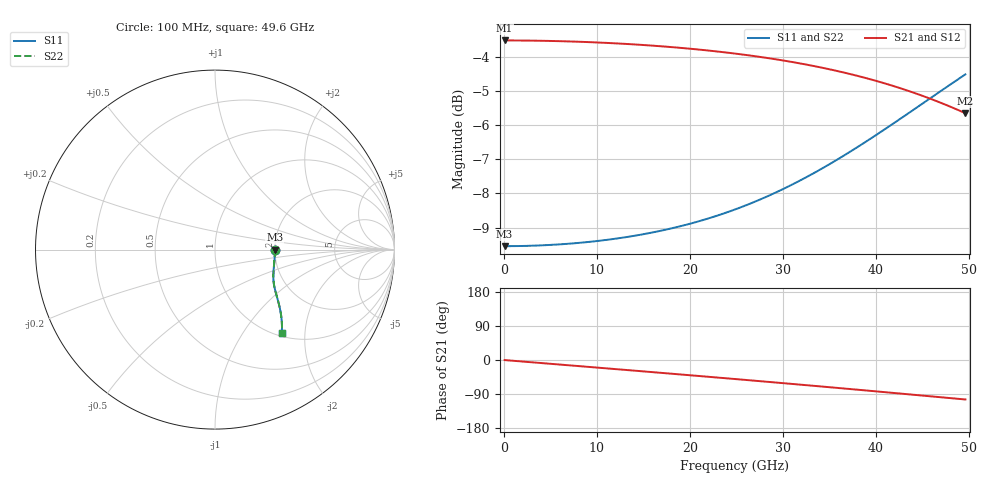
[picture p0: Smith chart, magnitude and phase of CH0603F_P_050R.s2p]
# GHz S RI R 50
! S-Parameters data
! Freq  reS11  imS11  reS21  imS21  reS12  imS12  reS22  imS22
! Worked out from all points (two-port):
!   100 points, 100 MHz to 49.6 GHz, reference 50 ohm
!   highest |S21| = -3.52 dB at 100 MHz (marker M1); lowest = -5.7 dB at 49.6 GHz (marker M2)
!   |S21| within 3 dB of the highest: start of sweep to end of sweep
!   lowest |S11| = -9.5 dB at 100 MHz (marker M3), VSWR 2.00, Z = 100 - j0.185 ohm
!   |S11| at or under -10 dB: nowhere
!   |S22| runs from -9.5 to -4.5 dB; largest |S21 - S12| = 0
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0.1  0.3333 -0.000824  0.6667 -0.00232  0.6667 -0.00232  0.3333 -0.000824
2.1  0.3331 -0.0173  0.6647 -0.0486  0.6647 -0.0486  0.3331 -0.0173
4.1  0.3326 -0.0336  0.6592 -0.0946  0.6592 -0.0946  0.3326 -0.0336
6.1  0.3317 -0.0498  0.6501 -0.1401  0.6501 -0.1401  0.3317 -0.0498
8.6  0.3303 -0.0696  0.6338 -0.1957  0.6338 -0.1957  0.3303 -0.0696
12.6  0.3278 -0.1002  0.5968 -0.2807  0.5968 -0.2807  0.3278 -0.1002
16.6  0.3257 -0.1294  0.547 -0.3589  0.547 -0.3589  0.3257 -0.1294
18.6  0.3252 -0.1435  0.5175 -0.3948  0.5175 -0.3948  0.3252 -0.1435
21.1  0.3253 -0.161  0.4767 -0.4363  0.4767 -0.4363  0.3253 -0.161
25.1  0.3277 -0.189  0.4032 -0.4934  0.4032 -0.4934  0.3277 -0.189
27.1  0.3301 -0.2036  0.3631 -0.5172  0.3631 -0.5172  0.3301 -0.2036
29.1  0.3333 -0.2187  0.321 -0.5375  0.321 -0.5375  0.3333 -0.2187
31.1  0.3373 -0.2348  0.2774 -0.554  0.2774 -0.554  0.3373 -0.2348
33.1  0.342 -0.252  0.2324 -0.5666  0.2324 -0.5666  0.342 -0.252
35.6  0.3486 -0.2755  0.175 -0.5765  0.175 -0.5765  0.3486 -0.2755
37.6  0.3541 -0.2963  0.1286 -0.5795  0.1286 -0.5795  0.3541 -0.2963
39.6  0.3596 -0.319  0.0824 -0.578  0.0824 -0.578  0.3596 -0.319
41.6  0.3647 -0.3438  0.0368 -0.5721  0.0368 -0.5721  0.3647 -0.3438
43.6  0.3689 -0.3707  -0.00752 -0.5617  -0.00752 -0.5617  0.3689 -0.3707
45.6  0.3719 -0.3998  -0.0501 -0.547  -0.0501 -0.547  0.3719 -0.3998
47.6  0.3731 -0.4309  -0.0903 -0.5283  -0.0903 -0.5283  0.3731 -0.4309
49.6  0.3722 -0.4638  -0.1277 -0.5058  -0.1277 -0.5058  0.3722 -0.4638
